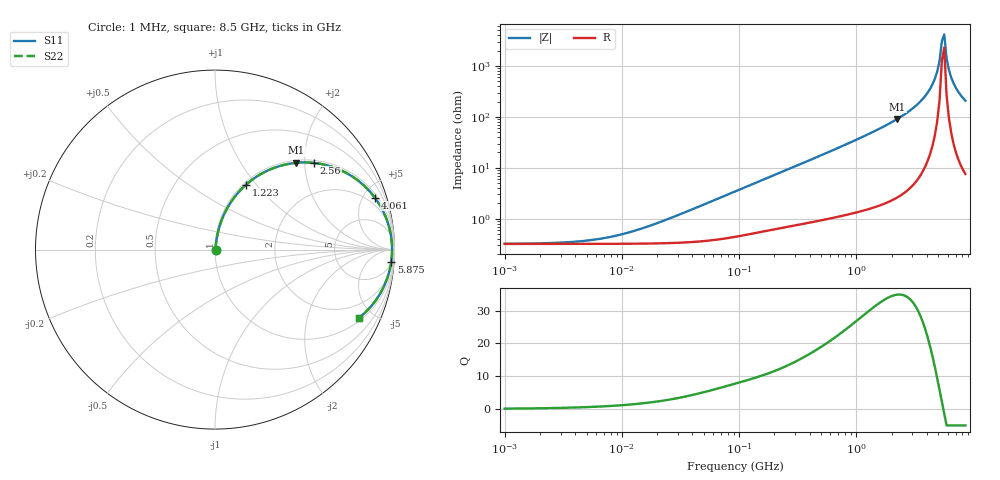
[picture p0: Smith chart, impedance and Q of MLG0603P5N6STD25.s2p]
! S-Parameter Data Generated by TDK Corporation
! Copyright(C) 2025 TDK Corporation.
! All Rights Reserved.
! TDK P/N: MLG0603P5N6STD25 (SMD / SMT Inductor (Coil))
! Property: L=5.6nH at 500MHz
! Size(LxWxT): 0.6x0.3x0.3mm
! Model Type: s2p (Touchstone File Format Version 1.0)
! Frequency: DC=Yes Start=1MHz Stop=8500MHz 198points Log-sweep
! Model Generated on Feb. 6, 2025
! Terms and conditions regarding TDK Simulation Models:
! 1)This simulation model is being provided solely for informational
!  purposes. Please refer to the specifications of the products in
!  terms of detailed characteristics of such products.
! 2)In no event shall TDK Corporation of any of its subsidiaries be
!  liable for any loss or damage arising, directly or indirectly,
!  from any information contained in this simulation model, including,
!  but not limited to loss or damages arising from any inaccuracies,
!  omissions or errors in connection with such information.
! 3)Any and all copyrights on this simulation model are owned by
!  TDK Corporation.  Duplication or redistribution of this simulation
!  model without prior written permission from TDK Corporation
!  is prohibited.
! 4)This simulation model is subject to any modification or change
!  without any prior notice.
! 5)Neither TDK Corporation nor any of its subsidiaries shall make any
!  warranty, express or implied, including but not limited to the
!  correctness, implied warranties of merchantability and fitness for
!  a particular purpose with respect to this simulation models.
! 6)The use of this simulation model shall be deemed to have consented
!  to the terms and conditions hereof.
! Port Assignments:
!  1 ---@@@--- 2
! Applicable Conditions:
!  Temperature = 25 degC
!  DC Bias Current = 0 A
!  Small Signal Operation
# Hz S MA R 50
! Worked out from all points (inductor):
!   197 points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, 1 MHz to 8.5 GHz, reference 50 ohm
!   read as one part in series: L = 5.96 nH near 27.76 MHz
!   highest Q = 34.9 at 2.229 GHz (marker M1), where L = 6.49 nH
!   self-resonance near 5.357 GHz
!   S11 on the Smith chart (normalised r, x): 1 MHz: 1.01, +0.00; 1.223 GHz: 1.03, +0.88; 2.56 GHz: 1.06, +2.22; 4.061 GHz: 1.28, +6.04; 5.875 GHz: 6, -28; 8.5 GHz: 1.15, -4.16
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1000000  0.003212 6.7  0.9968 -0.0  0.9968 -0.0  0.003212 6.7
4587603  0.003627 28.2  0.9968 -0.1  0.9968 -0.1  0.003627 28.2
9601846  0.004819 48.1  0.9968 -0.2  0.9968 -0.2  0.004819 48.1
2.10461e7  0.008526 67.0  0.9967 -0.5  0.9967 -0.5  0.008526 67.0
9.219544e7  0.03407 80.7  0.9951 -1.9  0.9951 -1.9  0.03407 80.7
4.229561e8  0.1464 78.3  0.9808 -8.4  0.9808 -8.4  0.1464 78.3
1.222927e9  0.3992 64.5  0.9034 -23.5  0.9034 -23.5  0.3992 64.5
1.940355e9  0.5951 51.8  0.7864 -36.5  0.7864 -36.5  0.5951 51.8
2.228565e9  0.6632 46.8  0.7296 -41.5  0.7296 -41.5  0.6632 46.8
2.559585e9  0.7332 41.2  0.6592 -47.1  0.6592 -47.1  0.7332 41.2
3.37643e9  0.8664 28.1  0.4711 -60.0  0.4711 -60.0  0.8664 28.1
4.061159e9  0.9366 18.0  0.31 -69.3  0.31 -69.3  0.9366 18.0
4.453958e9  0.9618 12.7  0.2204 -73.7  0.2204 -73.7  0.9618 12.7
4.884749e9  0.9788 7.2  0.1265 -76.7  0.1265 -76.7  0.9788 7.2
5.115526e9  0.9838 4.5  0.07873 -75.9  0.07873 -75.9  0.9838 4.5
5.357206e9  0.9865 1.7  0.03183 -64.0  0.03183 -64.0  0.9865 1.7
5.610304e9  0.9867 -1.1  0.02371 55.4  0.02371 55.4  0.9867 -1.1
5.87536e9  0.9845 -3.9  0.06972 75.2  0.06972 75.2  0.9845 -3.9
6.152938e9  0.9799 -6.7  0.1176 76.8  0.1176 76.8  0.9799 -6.7
6.748056e9  0.9638 -12.2  0.212 74.1  0.212 74.1  0.9638 -12.2
7.400733e9  0.9391 -17.6  0.3024 69.7  0.3024 69.7  0.9391 -17.6
8.5e9  0.8887 -25.3  0.4273 62.6  0.4273 62.6  0.8887 -25.3
